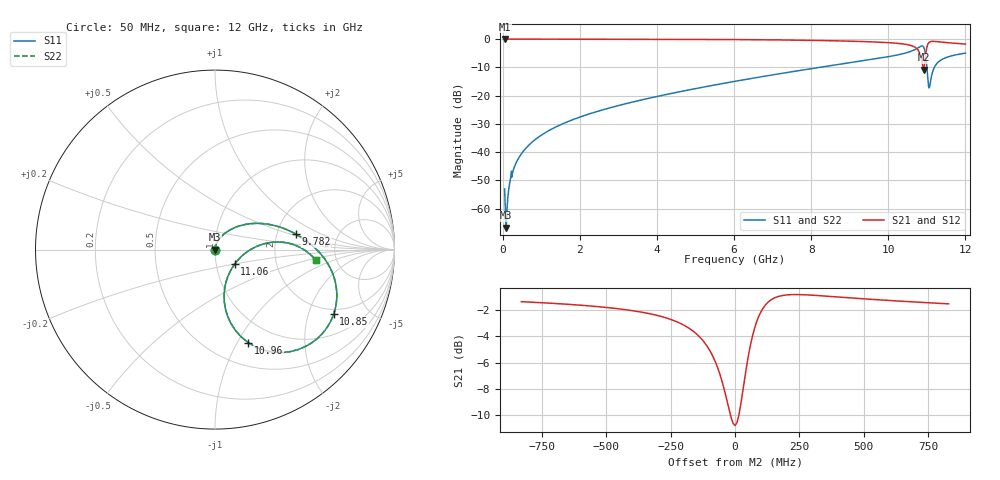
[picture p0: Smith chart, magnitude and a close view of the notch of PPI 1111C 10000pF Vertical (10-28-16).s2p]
# GHz S MA R 50
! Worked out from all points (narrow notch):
!   1601 points, 50 MHz to 12 GHz, reference 50 ohm
!   highest |S21| = 0.00 dB at 50 MHz (marker M1); lowest = -10.8 dB at 10.92 GHz (marker M2)
!   notch at M2: 10.6 dB deep, 139 MHz wide at half that depth
!   lowest |S11| = -66.8 dB at 87.34 MHz (marker M3), VSWR 1.00, Z = 50 - j0.00907 ohm
!   |S11| at or under -10 dB: start of sweep to 8.227 GHz; 11 GHz to 11.2 GHz (193.9 MHz wide, 1.75 % of centre)
!   |S22| runs from -66.8 to -2.4 dB; largest |S21 - S12| = 0
!   S11 on the Smith chart (normalised r, x): 50 MHz: 1.00, -0.00; 9.782 GHz: 2.56, +0.56; 10.85 GHz: 1.79, -2.95; 10.96 GHz: 0.75, -1.11; 11.06 GHz: 1.23, -0.20; 12 GHz: 3.48, -0.59
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0.05  0.00222 -80.7  0.9996 -0.2  0.9996 -0.2  0.00222 -80.7
0.08734375  0.0004589 -11.4  0.9995 -0.5  0.9995 -0.5  0.0004589 -11.4
0.1321563  0.001522 68.7  0.9995 -0.8  0.9995 -0.8  0.001522 68.7
0.1919063  0.003094 77.1  0.9994 -1.3  0.9994 -1.3  0.003094 77.1
0.2665938  0.004617 79.4  0.9993 -1.8  0.9993 -1.8  0.004617 79.4
0.5802812  0.01125 81.0  0.9989 -3.9  0.9989 -3.9  0.01125 81.0
1.147906  0.02293 78.9  0.9983 -7.8  0.9983 -7.8  0.02293 78.9
2.044156  0.04258 73.7  0.9972 -13.9  0.9972 -13.9  0.04258 73.7
4.038312  0.09759 60.5  0.9924 -28.0  0.9924 -28.0  0.09759 60.5
6.025  0.1788 45.8  0.9801 -43.1  0.9801 -43.1  0.1788 45.8
8.019156  0.3006 28.9  0.9486 -60.2  0.9486 -60.2  0.3006 28.9
9.781781  0.4601 10.7  0.8802 -78.4  0.8802 -78.4  0.4601 10.7
10.01331  0.4895 7.7  0.8632 -81.4  0.8632 -81.4  0.4895 7.7
10.61828  0.6191 -5.5  0.7577 -93.0  0.7577 -93.0  0.6191 -5.5
10.84981  0.7523 -28.4  0.4788 -102.0  0.4788 -102.0  0.7523 -28.4
10.91703  0.7246 -50.2  0.288 -70.8  0.288 -70.8  0.7246 -50.2
10.96184  0.5507 -70.3  0.4844 -40.1  0.4844 -40.1  0.5507 -70.3
11.00666  0.2901 -79.8  0.7422 -47.5  0.7422 -47.5  0.2901 -79.8
11.05894  0.1361 -36.3  0.8731 -59.8  0.8731 -59.8  0.1361 -36.3
11.14856  0.2615 6.2  0.9122 -71.9  0.9122 -71.9  0.2615 6.2
11.33528  0.4118 5.0  0.8899 -82.1  0.8899 -82.1  0.4118 5.0
12  0.5638 -5.9  0.8163 -95.0  0.8163 -95.0  0.5638 -5.9
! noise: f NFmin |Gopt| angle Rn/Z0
0.05  0.0004129  0.8785  0.2827  0.0007346
1.372  0.004377  0.7141  7.619  0.003008
2.701  0.007274  0.6731  14.83  0.004217
4.031  0.009939  0.6535  21.82  0.005274
5.36  0.01258  0.6464  28.55  0.006349
6.682  0.01532  0.6486  34.96  0.00756
8.012  0.01842  0.6598  41.12  0.009123
9.341  0.02274  0.6869  47.1  0.01193
10.67  0.06366  0.8641  54.42  0.07965
12  0.03157  0.7288  58.61  0.01776
